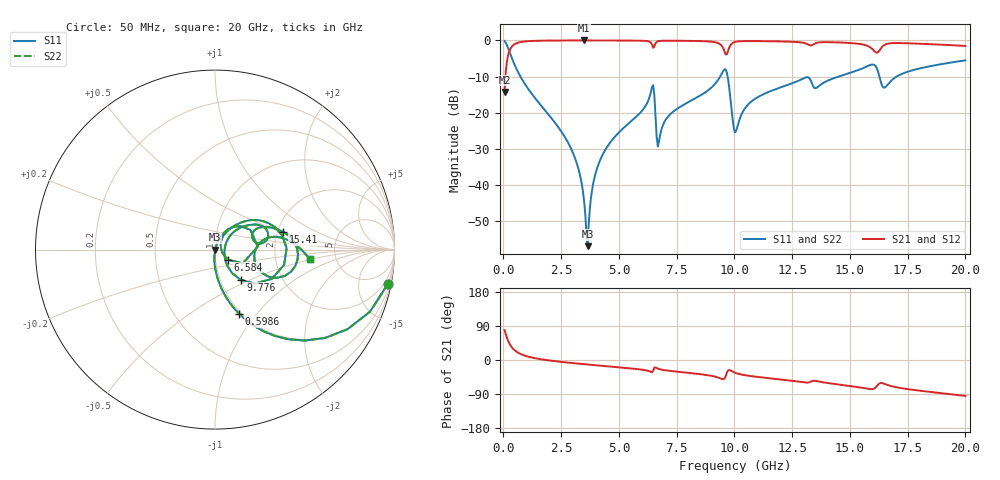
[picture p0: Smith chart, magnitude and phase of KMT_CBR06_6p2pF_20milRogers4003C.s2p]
! Data measured by Modelithics Inc. support@modelithics.com 813-866-6335
! KEMET CBR0603 6.2pF, Pad Width= 0.851mm, Pad Length= 0.64mm, Pad Gap= 0.62mm, 20mil Rogers 4003C substrate Data, January 2022
# hz S ma R 50
! 2 Port Network Data from SP1.SP block
! freq  magS11  angS11  magS21  angS21  magS12  angS12  magS22  angS22
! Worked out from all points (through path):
!   401 points, 50 MHz to 20 GHz, reference 50 ohm
!   highest |S21| = -0.01 dB at 3.491 GHz (marker M1); lowest = -14.3 dB at 50 MHz (marker M2)
!   group delay of S21, straight-line fit = 14.6 ps
!   lowest |S11| = -57.0 dB at 3.641 GHz (marker M3), VSWR 1.00, Z = 50.1 + j0.012 ohm
!   |S11| at or under -10 dB: 733.5 MHz to 9.384 GHz (8.65 GHz wide, 171 % of centre); 9.705 GHz to 14.53 GHz (4.823 GHz wide, 39.8 % of centre); 16.28 GHz to 17.03 GHz (750.3 MHz wide, 4.51 % of centre)
!   |S22| runs from -57.0 to -0.2 dB; largest |S21 - S12| = 0
!   S11 on the Smith chart (normalised r, x): 50 MHz: 1, -10; 598.6 MHz: 0.97, -0.82; 6.584 GHz: 1.15, -0.13; 9.776 GHz: 1.25, -0.44; 15.41 GHz: 2.15, +0.50; 20 GHz: 3.18, -0.46
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5e7  0.9812 -11.3  0.1929 78.7  0.1929 78.7  0.9812 -11.3
2.495e8  0.7121 -45.4  0.7015 44.6  0.7015 44.6  0.7121 -45.4
5.98625e8  0.3824 -69.4  0.9233 20.5  0.9233 20.5  0.3824 -69.4
2.74325e9  0.0412 -94.9  0.9979 -6.6  0.9979 -6.6  0.0412 -94.9
3.391625e9  0.0102 -93.1  0.9985 -10.5  0.9985 -10.5  0.0102 -93.1
3.491375e9  0.005987 -88.3  0.9985 -11.0  0.9985 -11.0  0.005987 -88.3
3.641e9  0.00141 4.9  0.9985 -11.9  0.9985 -11.9  0.00141 4.9
3.94025e9  0.01249 70.0  0.9984 -13.5  0.9984 -13.5  0.01249 70.0
4.439e9  0.0316 71.0  0.9978 -16.2  0.9978 -16.2  0.0316 71.0
6.434e9  0.2258 29.3  0.8725 -32.3  0.8725 -32.3  0.2258 29.3
6.583625e9  0.09039 -38.2  0.9137 -19.7  0.9137 -19.7  0.09039 -38.2
6.73325e9  0.03983 37.2  0.9799 -23.8  0.9799 -23.8  0.03983 37.2
7.182125e9  0.0922 58.5  0.9907 -28.5  0.9907 -28.5  0.0922 58.5
9.52625e9  0.3826 11.9  0.763 -50.5  0.763 -50.5  0.3826 11.9
9.775625e9  0.2199 -49.7  0.7939 -26.4  0.7939 -26.4  0.2199 -49.7
1.0025e10  0.05326 -7.3  0.9516 -33.6  0.9516 -33.6  0.05326 -7.3
1.10225e10  0.1645 42.4  0.9781 -44.8  0.9781 -44.8  0.1645 42.4
1.336662e10  0.2493 7.5  0.8613 -55.5  0.8613 -55.5  0.2493 7.5
1.54115e10  0.3935 14.4  0.8947 -72.0  0.8947 -72.0  0.3935 14.4
1.62095e10  0.3775 -24.7  0.6832 -65.7  0.6832 -65.7  0.3775 -24.7
1.670825e10  0.26 9.7  0.9092 -67.5  0.9092 -67.5  0.26 9.7
2e10  0.5295 -5.7  0.8383 -94.7  0.8383 -94.7  0.5295 -5.7
